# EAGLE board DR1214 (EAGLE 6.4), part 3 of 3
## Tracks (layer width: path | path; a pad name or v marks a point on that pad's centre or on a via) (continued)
VDD_3V3  (via drill 0.15 layers 1-2, 0.15 layers 15-16, 0.25, 0.25 layers 2-15,  (continued)
  Bottom 0.305: IC4.8 76.08,16.43 76,16.5 | R2.2 38.1,56.5 v38,56.4 | R50.1 44.65,30.95 v44.4,31.2 | C138.1 27.25,29.6 v27,29.6 L17.2 | R108.2 R109.2 v58,56.4
  Bottom 0.406: R28.1 R27.1 31.05,5.7 29.85,6.9 | 10.5,37.5 v13.5,34.5 | R72.2 77.4,13.4 v77.75,13.75 | v77.5,16.25 77.25,16.5 76,16.5 76,17.4 R129.2 | R61.2 30.46,44.44 30.8,44.77 IC1.4 IC1.3 34.66,45.89 IC2.5 R1.2 34.92,44.75 34.92,44.13 35.24,43.81 37.15,43.81 37.47,44.13 C1.1 38.54,46.34 38.8,46.6 v38.8,47.8 | R78.2 92.5,17.85 | 92.5,17.85 R58.2 | C67.1 92.4,17.95 92.5,17.85 | v47,56.4 R132.2 | R12.1 51.2,46 v50.2,47 | D2.2 v47.81,46.79 v47.8,46.8 | C26.1 C34.1 C139.1 | C139.1 29.85,13.96 ETH.3 | C139.1 C140.1 29.85,6.9 | 29.85,6.9 R25.1 | v32.6,33 33.17,33.57 R68.1 32.95,34.04 L6.2 | v44,20.8 44,23.25 L8.2
  Bottom 0.61: v10,38 10.5,37.5 | R7.2 R9.2 R5.2 R6.2 29.15,23.2 v27.2,23.2 | ETH.3 29.23,15.85 ETH.4 | C9.2 R129.2 | R72.2 78.4,12.75 | 78.4,12.75 R71.2 | v77.4,11.6 78.2,12.4 78.2,12.55 78.4,12.75 | C68.1 93.03,42.8 v94.4,42.8 v95.2,42.8 | v91.4,24 v92.4,24 | v64.2,7.6 64.15,7.55 R73.2
  other vias: 62.81,32.4 11,39
  pour Top (isolate 0.254): 8,44 11,44 12.5,42.5 12.5,40 9.75,37.25 9,37.25 9,38 8,39
  pour Route14 (isolate 0.2): 8.8,37.6 8.8,42.4 10.4,44 14.4,44 15.2,44.8 15.2,56 16.8,57.6 67.2,57.6 68,58.4 72.2,58.4 72.8,57.8 72.8,56 72.2,55.4 69,55.4 59.2,45.6 47.2,45.6 45.6,47.2 37.2,47.2 35.2,49.2 19.8,49.2 18.2,47.6 18.2,36.2 23.2,31.2 28.2,31.2 30.4,33.4 43,33.4 43.6,32.8 43.6,30.8 43.2,30.4 37.8,30.4 36.8,29.4 36.8,23 38.2,21.6 57.4,21.6 58.4,22.6 58.4,30.2 60.4,32.2 62.2,32.2 64,30.4 68,30.4 68.4,30.8 68.4,32.4 69.2,32.4 71.2,34.4 84.8,34.4 86.6,36.4 86.6,39.4 91.2,43.8 96.2,43.8 98,42 98,31.25 99.4,29.85 101.7,29.85 102.95,28.6 102.95,26.7 101.45,25.2 97.2,25.2 95.2,23.2 82.4,23.2 78.4,19.2 78.4,5.6 76.8,4 65.6,4 61.6,8 50.4,8 49.6,8.8 49.6,16 46.6,19 40.8,19 35.2,13.4 29,13.4 15.2,27.2 15.2,28.8 12.8,31.2 12.8,35 11.2,36.8 9.6,36.8
VDD_5V  (via drill 0.25, 0.5)
  Top 0.305: 13,21.73 IC5.6 | IC5.1 9.65,25.08 9.5,25.23
  Top 0.406: v13.5,21.73 13,21.73 | 9.5,25.23 v10,25.23 | EXT.15 EXT.13
  Top 0.61: 9.5,25.23 9.5,27.83 | 9.5,27.83 9.6,27.73 C11.1 | EXT.13 74.54,5.54 v74.6,5.6 v75.4,5.6 | 9.5,27.83 L16.2
  Route14 0.61: 12,28 11.2,28 | 11.2,28 11.2,29.83 | 11.2,28 11.2,26.2 10.23,25.23 v10,25.23 | v75.4,5.6 v74.6,5.6
  Route14 1.27: v74.6,5.6 71.4,2.4 58.6,2.4 58,1.8 51.2,1.8 50.6,2.4 42.4,2.4 | 41.6,2.4 39.6,2.4 39,1.8 36.8,1.8 36.2,2.4 32.8,2.4 31.2,4 31.2,6.7 24.8,13.1 24.8,15.2 12,28 | v42.4,1.6 42.4,2.4 | 42.4,2.4 41.6,2.4 | 41.6,2.4 v41.6,1.6
  Bottom 0.406: v13.5,21.73 13,21.73 10,24.73 v10,25.23
  Bottom 0.61: 40,1.6 v41.6,1.6 v42.4,1.6 43.1,1.6
  Bottom 0.612: C127.1 44.35,2.9 U5.1 43.45,1.95 43.1,1.6 | C126.2 39.6,2 40,1.6
  other vias: 10.8,25.83 11,29.83
  pour Top (isolate 0.305): 8,31 10.5,31 12.5,29 12.5,27 9.75,24.25 9.25,24.25 9.25,25.25 8,26.5
  pour Route14 (isolate 0.2): 9.6,30.4 12,30.4 14,28.4 14,22 13.6,21.6 12.8,21.6 8.8,25.6 8.8,29.6
VDD_EMC  (via drill 0.15 layers 1-2, 0.15 layers 15-16, 0.25, 0.25 layers 2-15)
  Top 0.127: IC7.N11 v64.8,36 | IC7.N10 v65.6,36 | v66.4,36 v66.39,36 IC7.N9 | IC7.N8 v67.2,36 | v67.2,36 IC7.N7 v67.61,36.39 v68,36 | v68,33.61 IC7.K6 | IC7.K7 v68,34.4 IC7.L6 | IC7.M8 v67.2,36 | IC10.K9 87.6,43.6 88.2,43.6 v88.6,44 | v88.6,51.2 IC10.A9 | IC10.C9 v88.6,49.6 | IC10.E9 v88.6,48 | IC10.F9 v88.6,47.2 | IC10.D1 80,48.8 v78.2,50.6 | IC10.B1 80.4,50.8 v80.4,51.6 | IC10.A7 v85.6,52.2 | v68,32.8 v68,32.81 IC7.J6 | v68,35.2 IC7.M6
  Top 0.406: LR5.2 66.9,51.5 v67.2,51.2 | v67.2,51.2 v67.2,50.4 v68,50.4 v68,51.2 v67.2,51.2
  Route2 0.127: v67.6,33.2 v68,32.8 | v68.4,34 v68,34.4 | v68.4,34.8 v68,35.2 | v66.8,36.4 v67.2,36 | v66,36.4 v66.4,36 | v65.2,36.4 v65.6,36 | v64.4,36.4 v64.8,36 | v68,36 v68.4,35.6 | v68.4,33.2 v68.01,33.6 v68,33.61 | v78.2,50.6 v77.6,50.6 | v80.4,51.6 v79.4,51.6
  Route14 0.127: v64.4,36.4 v65.2,36.4 v66,36.4 v66.8,36.4 v67.6,36.4 | v68.4,34.8 v68.4,34 v68.4,33.2 v67.6,33.2
  Route14 0.406: v68,51.2 68.8,51.2 | 68.8,51.2 73.8,51.2 74.8,50.2 77.2,50.2 v77.6,50.6 v78.6,51.6 v79.4,51.6 83,51.6 83.6,52.2 v85.6,52.2 88,52.2 88.6,51.6 v88.6,51.2 v88.6,49.6 v88.6,48 v88.6,47.2 v88.6,44 | 68.8,51.2 69.6,50.4 69.6,37.6 68.4,36.4 v67.6,36.4 67.6,35.6 v68.4,34.8 | v83.4,35.4 83.4,38.2
  Route14 0.5: 83.4,38.2 83.4,40.2 IC10.K9 v88.6,44
  Route15 0.127: v64.4,36.4 v64.8,36.8 | v65.2,36.4 v65.6,36.8 | v66,36.4 v66.4,36.8 | v66.8,36.4 v67.2,36.8 | v67.6,36.4 v68,36.8 | v68.4,35.6 v68.8,35.2 | v68.4,34.8 v68.8,34.4 | v68.4,34 v68.8,33.6 | v68.4,33.2 v68.8,32.8 | v79.4,51.6 v78.6,51.6 | v77.6,50.6 v77,50.6
  Bottom 0.127: C13.1 69,34.6 v68.8,34.4 | C15.1 69,33.4 v68.8,33.6 | C12.1 69.4,32.2 v68.8,32.8 | v77,50.6 76.8,50.8 C79.1 | C78.1 v78.6,51.6 | C16.1 69.4,35.8 v68.8,35.2 | C18.1 66.2,37 v66.4,36.8 | C25.1 67.4,37 v67.2,36.8 | C29.1 68.6,37.4 v68,36.8 | C17.1 65,37.4 v65.6,36.8 | C30.1 64.15,37.45 v64.8,36.8
  Bottom 0.254: R80.2 C77.1 | C83.1 v88.6,51.2 | C82.1 89.4,48.8 v88.6,48 | C81.1 v88.6,47.2 | C80.1 89.4,44.8 v88.6,44
  Bottom 0.406: R80.2 74.6,37.55 74.6,35.95 | v83.4,35.4 77,35.4 76.2,36.2 74.85,36.2 74.6,35.95 | 74.6,35.95 C14.1
  pour Route14 (isolate 0.2): 64.4,38.8 64.4,36.4 65.2,35.6 67,35.6 67.6,35 67.6,33.2 67.8,33 68.8,33 71,35.2 84.6,35.2 85.8,36.6 85.8,39.6 89.6,43.2 89.6,52 87.2,54.4 69.6,54.4 66.4,51.2 66.4,40.8
VDD_ETH  (via drill 0.25)
  Route3 0.256: v41.3,31.4 41.3,31 41.8,30.5 41.8,26.5 v41.7,26.4
  Route14 0.256: v38.1,31.7 41,31.7 v41.3,31.4
  Bottom 0.256: U201.26 37.62,31.22 v38.1,31.7 | v41.3,31.4 42.05,31.4 C135.1 | U201.1 41.6,24.98 | 41.6,24.98 42.48,24.98 C136.1 | v41.7,26.4 41.7,25.08 41.6,24.98
  Bottom 0.406: L8.1 42.35,24.85 C136.1
VDD_IN  (via drill 0.6)
  Top 0.305: IC5.4 9,22.23 8.5,21.73 | IC12.4 IC12.5 9,34.5
  Top 0.61: 8.5,21.73 7.65,21.73 C8.1 6.35,21.58 v6,21.23 v6,19.73 | v17.4,18 v17.4,19.4 | 9,34.5 7.65,34.5 C118.1 6.35,34.35 v6,34 v6,32.5
  Bottom 0.61: v6,21.23 v6,19.73 15.67,19.73 v17.4,18 | v17.4,18 v17.4,19.4 16.3,20.5 12,20.5 6,26.5 v6,32.5 v6,34 | v17.4,18 v17.4,16.6
  pour Top (isolate 0.254): 14,20 16.4,20 18.2,22 19.5,22 19.5,16 14,16
  pour Route14 (isolate 0.2): 4,34.4 4.8,35.2 6.4,35.2 7.2,34.4 7.2,25.8 12.4,20.6 17.4,20.6 18.2,19.8 18.2,16.8 17.4,16 12,16 9.6,18.4 5.6,18.4 4,20
VDD_USB  (via drill 0.25)
  Top 0.254: R149.2 R144.2 R143.2 R147.2 62.65,13.5 R16.2
  Top 0.256: v63.6,13.05 63.55,13 R147.2 | v53.6,9.45 53.45,9.3 C122.1 | IC13.24 57.25,9.05 v57.2,9 57.6,8.6 C120.1 | L5.2 53.65,16.75 v53.7,16.8 53.8,16.9 53.8,17.8 54.15,18.15 R35.2 R17.2 | IC13.20 55.25,9.05 v55.2,9
  Route3 0.256: v63.6,13.05 62.2,13.05 58.8,16.45 54.05,16.45 v53.7,16.8 53.6,16.7 v53.6,9.45 54.75,9.45 v55.2,9 v57.2,9
VDDA
  Bottom 0.254: 61.85,46.3 L1.1 62.4,46.85 D1.3

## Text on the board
Top: 1
Route2: 2
Route3: 3
Route14: 4
Route15: 5
Bottom: 6
tPlace: k | k | k | k | k | k | SEMICONDUCTORS | Data: | Address: | DR1214 0V1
